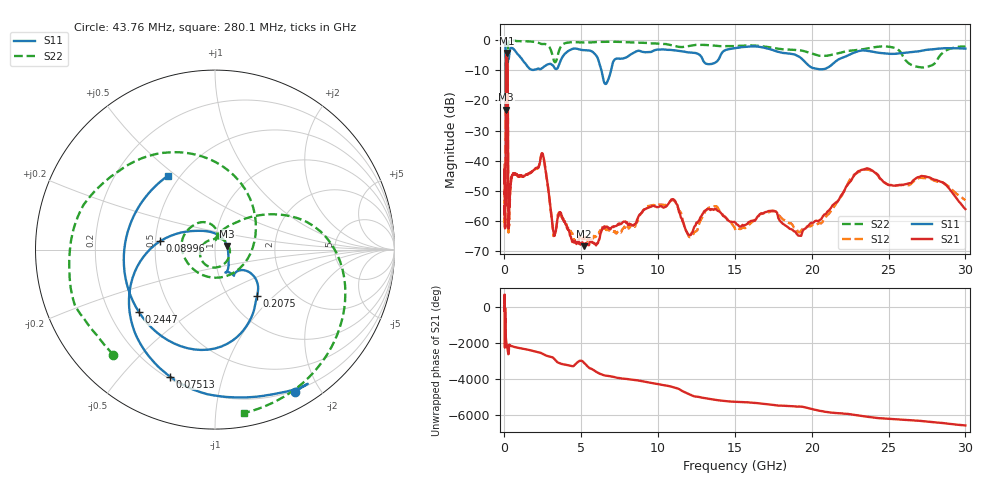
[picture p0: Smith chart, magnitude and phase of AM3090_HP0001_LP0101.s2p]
! Date/Time: Thu, Feb 28, 2019 1:54 PM
! Network Analyzer: Agilent Technologies E8364B Rev: A.07.50.67
! Sweep from 0.010 to 30.000 GHz, 1601 Points, Sweep Type: LOG
! Power Supply: 5.023 V, 0.002 A
# Hz S DB R 50
!freq MagS11 AngS11 MagS21 AngS21 MagS12 AngS12 MagS22 AngS22
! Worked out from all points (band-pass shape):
!   1601 points, 10 MHz to 30 GHz, reference 50 ohm
!   highest |S21| = -4.31 dB at 142.6 MHz (marker M1); lowest = -68.3 dB at 5.18 GHz (marker M2)
!   |S21| within 3 dB of the highest: 99.68 MHz to 201.2 MHz (101.6 MHz wide, 67.5 % of centre)
!   lowest |S11| = -23.1 dB at 98.44 MHz (marker M3), VSWR 1.15, Z = 57.2 + j2.36 ohm
!   |S11| at or under -10 dB: 89.82 MHz to 202.6 MHz (112.7 MHz wide, 77.1 % of centre); 6.309 GHz to 6.936 GHz (627.8 MHz wide, 9.48 % of centre)
!   |S22| runs from -25.6 to -0.2 dB; largest |S21 - S12| = 0.011
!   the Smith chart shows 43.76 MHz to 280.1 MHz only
!   S11 on the Smith chart (normalised r, x): 43.76 MHz: 0.18, -1.69; 75.13 MHz: 0.21, -0.69; 89.96 MHz: 0.53, +0.06; 207.5 MHz: 1.35, -0.79; 244.7 MHz: 0.33, -0.33; 280.1 MHz: 0.43, +0.47
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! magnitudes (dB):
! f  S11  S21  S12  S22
! 10 MHz  -0.3  -47.4  -40.9  -0.6
! 38.04 MHz  -0.5  -60.9  -59.8  -1.4
! 43.76 MHz  -0.8  -59.7  -58.4  -1.8
! 75.13 MHz  -2.5  -45.9  -46.2  -4.5
! 89.96 MHz  -10.2  -15.3  -15.3  -15.9
! 98.44 MHz  -23.1  -7.8  -7.7  -14.4
! 142.6 MHz  -15.5  -4.3  -4.3  -22.3
! 144.7 MHz  -15.4  -4.3  -4.3  -22.0
! 207.5 MHz  -9.2  -8.9  -8.9  -15.4
! 244.7 MHz  -5.2  -54.0  -54.8  -1.6
! 280.1 MHz  -6.2  -60.7  -62.9  -0.7
! 550.5 MHz  -2.9  -44.4  -44.3  -0.2
! 2.084 GHz  -9.7  -42.3  -42.5  -0.8
! 2.533 GHz  -8.9  -38.5  -38.5  -1.3
! 3.236 GHz  -9.1  -64.5  -64.9  -7.1
! 5.18 GHz  -3.4  -68.3  -65.7  -0.8
! 6.619 GHz  -14.5  -61.8  -63.0  -0.6
! 7.926 GHz  -5.8  -60.6  -61.3  -0.7
! 10.76 GHz  -3.3  -53.6  -53.5  -1.6
! 19.22 GHz  -5.6  -64.8  -63.7  -3.4
! 23.48 GHz  -3.5  -42.7  -42.9  -2.9
! 30 GHz  -2.9  -56.0  -53.0  -2.2
